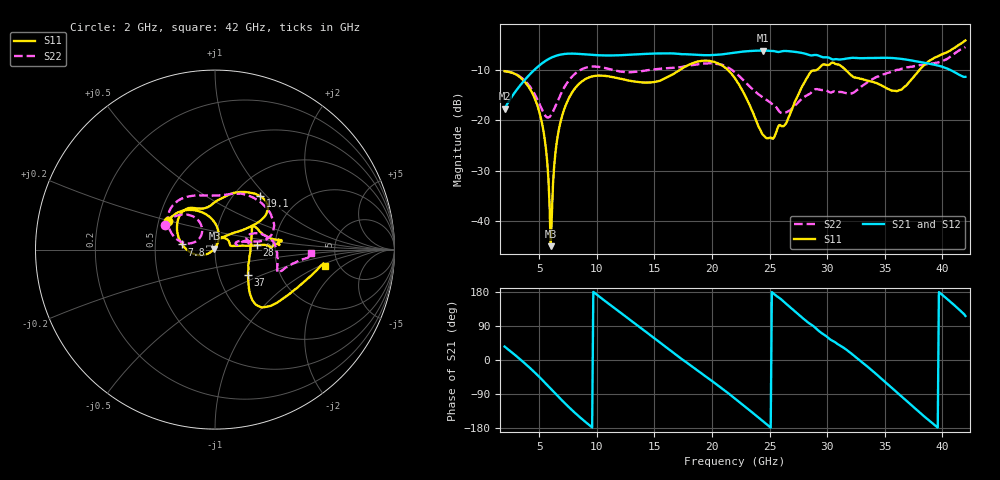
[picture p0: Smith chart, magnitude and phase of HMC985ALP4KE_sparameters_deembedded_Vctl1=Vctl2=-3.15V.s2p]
!s2p File: Measurements: S11, S21, S12, S22
# GHz S dB R 50.0
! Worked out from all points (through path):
!   401 points, 2 GHz to 42 GHz, reference 50 ohm
!   highest |S21| = -6.14 dB at 24.4 GHz (marker M1); lowest = -17.7 dB at 2 GHz (marker M2)
!   lowest |S11| = -44.9 dB at 6 GHz (marker M3), VSWR 1.01, Z = 49.7 + j0.476 ohm
!   |S11| at or under -10 dB: start of sweep to 17.21 GHz; 21.38 GHz to 29.06 GHz (7.679 GHz wide, 30.4 % of centre); 31.6 GHz to 38.01 GHz (6.402 GHz wide, 18.4 % of centre)
!   |S22| runs from -19.4 to -5.5 dB; largest |S21 - S12| = 0.00053
!   S11 on the Smith chart (normalised r, x): 2 GHz: 0.56, +0.20; 7.8 GHz: 0.69, +0.04; 19.1 GHz: 1.31, +0.92; 28 GHz: 1.61, +0.08; 37 GHz: 1.38, -0.41; 42 GHz: 3.91, -1.17
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2  -10.23 149.0  -17.66 35.4  -17.67 35.4  -10.22 154.0
4.8  -16.73 89.5  -9.51 -38.4  -9.51 -38.4  -15.61 119.1
5.5  -24.01 70.6  -8.27 -59.8  -8.27 -59.8  -18.95 131.6
6  -44.91 122.6  -7.61 -75.6  -7.61 -75.6  -19.03 153.6
6.7  -21.91 -157.4  -7.02 -97.8  -7.02 -97.8  -15.62 167.7
7.8  -14.66 171.1  -6.75 -130.8  -6.75 -130.8  -11.45 157.7
8.7  -12.28 150.6  -6.84 -155.4  -6.84 -155.4  -9.84 144.3
10.5  -11.11 126.3  -7.10 160.8  -7.10 160.8  -9.49 119.5
12.5  -11.95 114.7  -7.02 114.9  -7.02 114.9  -10.42 94.2
15.4  -12.18 95.9  -6.71 48.0  -6.71 48.0  -9.76 72.7
17.1  -10.16 76.9  -6.78 8.6  -6.78 8.6  -9.48 67.8
19.1  -8.19 49.7  -7.04 -35.6  -7.04 -35.5  -8.80 48.2
22  -11.64 32.4  -6.53 -101.8  -6.53 -101.8  -10.46 11.9
24.4  -22.77 64.9  -6.14 -160.8  -6.14 -160.8  -15.40 16.3
26.3  -20.94 14.4  -6.22 152.2  -6.22 152.2  -18.45 17.3
28  -12.55 5.9  -6.71 107.5  -6.71 107.5  -15.35 15.5
28.7  -10.13 1.6  -7.09 91.7  -7.10 91.7  -14.24 13.3
32.4  -11.47 23.0  -7.59 9.5  -7.58 9.5  -14.31 22.1
35.4  -13.85 8.7  -7.59 -67.8  -7.58 -67.9  -10.49 13.8
37  -12.72 -37.3  -7.97 -111.1  -7.98 -111.2  -9.46 4.0
39.4  -7.48 -49.3  -9.00 -173.3  -9.00 -173.3  -8.56 -19.9
42  -4.14 -8.5  -11.35 116.1  -11.35 116.1  -5.45 -2.3
